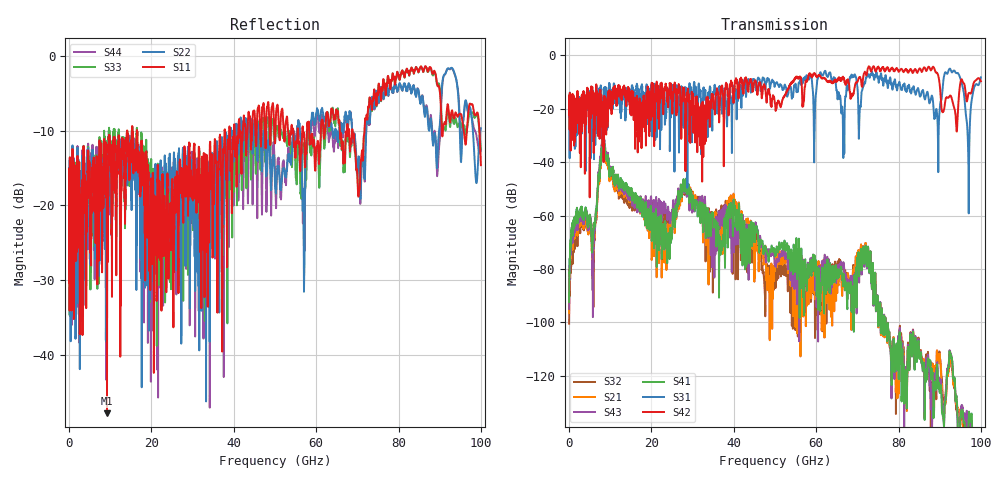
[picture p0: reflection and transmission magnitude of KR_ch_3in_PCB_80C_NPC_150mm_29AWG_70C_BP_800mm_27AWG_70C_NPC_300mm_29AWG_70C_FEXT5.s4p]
# GHz S RI R 45
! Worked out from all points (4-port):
!   4000 points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, 25 MHz to 100 GHz, reference 45 ohm
!   strongest paths, dB at 25 MHz, 25.02 GHz, 50.02 GHz, 75.03 GHz, 100 GHz:
!     S42: -20.7, -17.7, -18.0, -4.4, -9.7
!     S31: -20.7, -11.5, -11.2, -8.1, -8.3
!     S41: -92.4, -66.3, -75.2, -94.1, -159.8
!     S43: -95.0, -58.4, -78.9, -94.0, -173.0
!     S21: -96.5, -62.7, -75.5, -94.2, -169.1
!     S32: -100.5, -62.4, -81.9, -94.3, -179.4
!   lowest |S11| = -47.8 dB at 9.225 GHz (marker M1), VSWR 1.01, Z = 45.1 + j0.337 ohm
!   |S11| at or under -10 dB: start of sweep to 14.12 GHz; 16.48 GHz to 37.76 GHz (21.29 GHz wide, 78.5 % of centre); 68.85 GHz to 71.75 GHz (2.901 GHz wide, 4.13 % of centre)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
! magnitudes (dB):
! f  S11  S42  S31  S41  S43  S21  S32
! 25 MHz  -16.4  -20.7  -20.7  -92.4  -95.0  -96.5  -100.5
! 9.225 GHz  -47.8  -26.2  -24.3  -38.6  -37.4  -39.9  -38.6
! 24.05 GHz  -21.8  -18.3  -15.5  -68.3  -56.7  -65.3  -60.8
! 28.05 GHz  -12.3  -17.5  -12.3  -49.9  -50.7  -50.5  -51.5
! 92.55 GHz  -8.9  -15.1  -5.1  -111.7  -111.3  -113.2  -112.8
! 96.92 GHz  -7.7  -14.7  -36.8  -141.2  -142.4  -146.2  -151.6
! 100 GHz  -14.6  -9.7  -8.3  -159.8  -173.0  -169.1  -179.4
